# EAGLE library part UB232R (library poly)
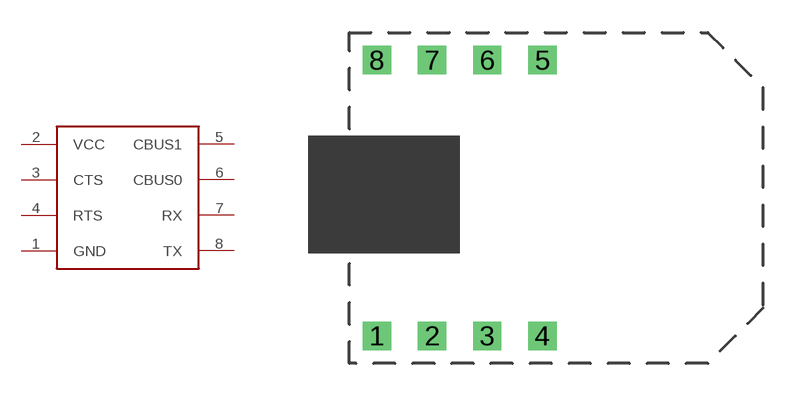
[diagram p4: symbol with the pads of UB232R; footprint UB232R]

Designator prefix -

## UB232R  [UB232R]
1  GND  pwr
2  VCC  sup
3  CTS
4  RTS
5  CBUS1
6  CBUS0
7  RX  in
8  TX  out

## Footprint UB232R (pad centres in mm)
drill 0.8 square: 1 -7.62,-6.35; 2 -5.08,-6.35; 3 -2.54,-6.35; 4 0,-6.35; 5 0,6.35; 6 -2.54,6.35; 7 -5.08,6.35; 8 -7.62,6.35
